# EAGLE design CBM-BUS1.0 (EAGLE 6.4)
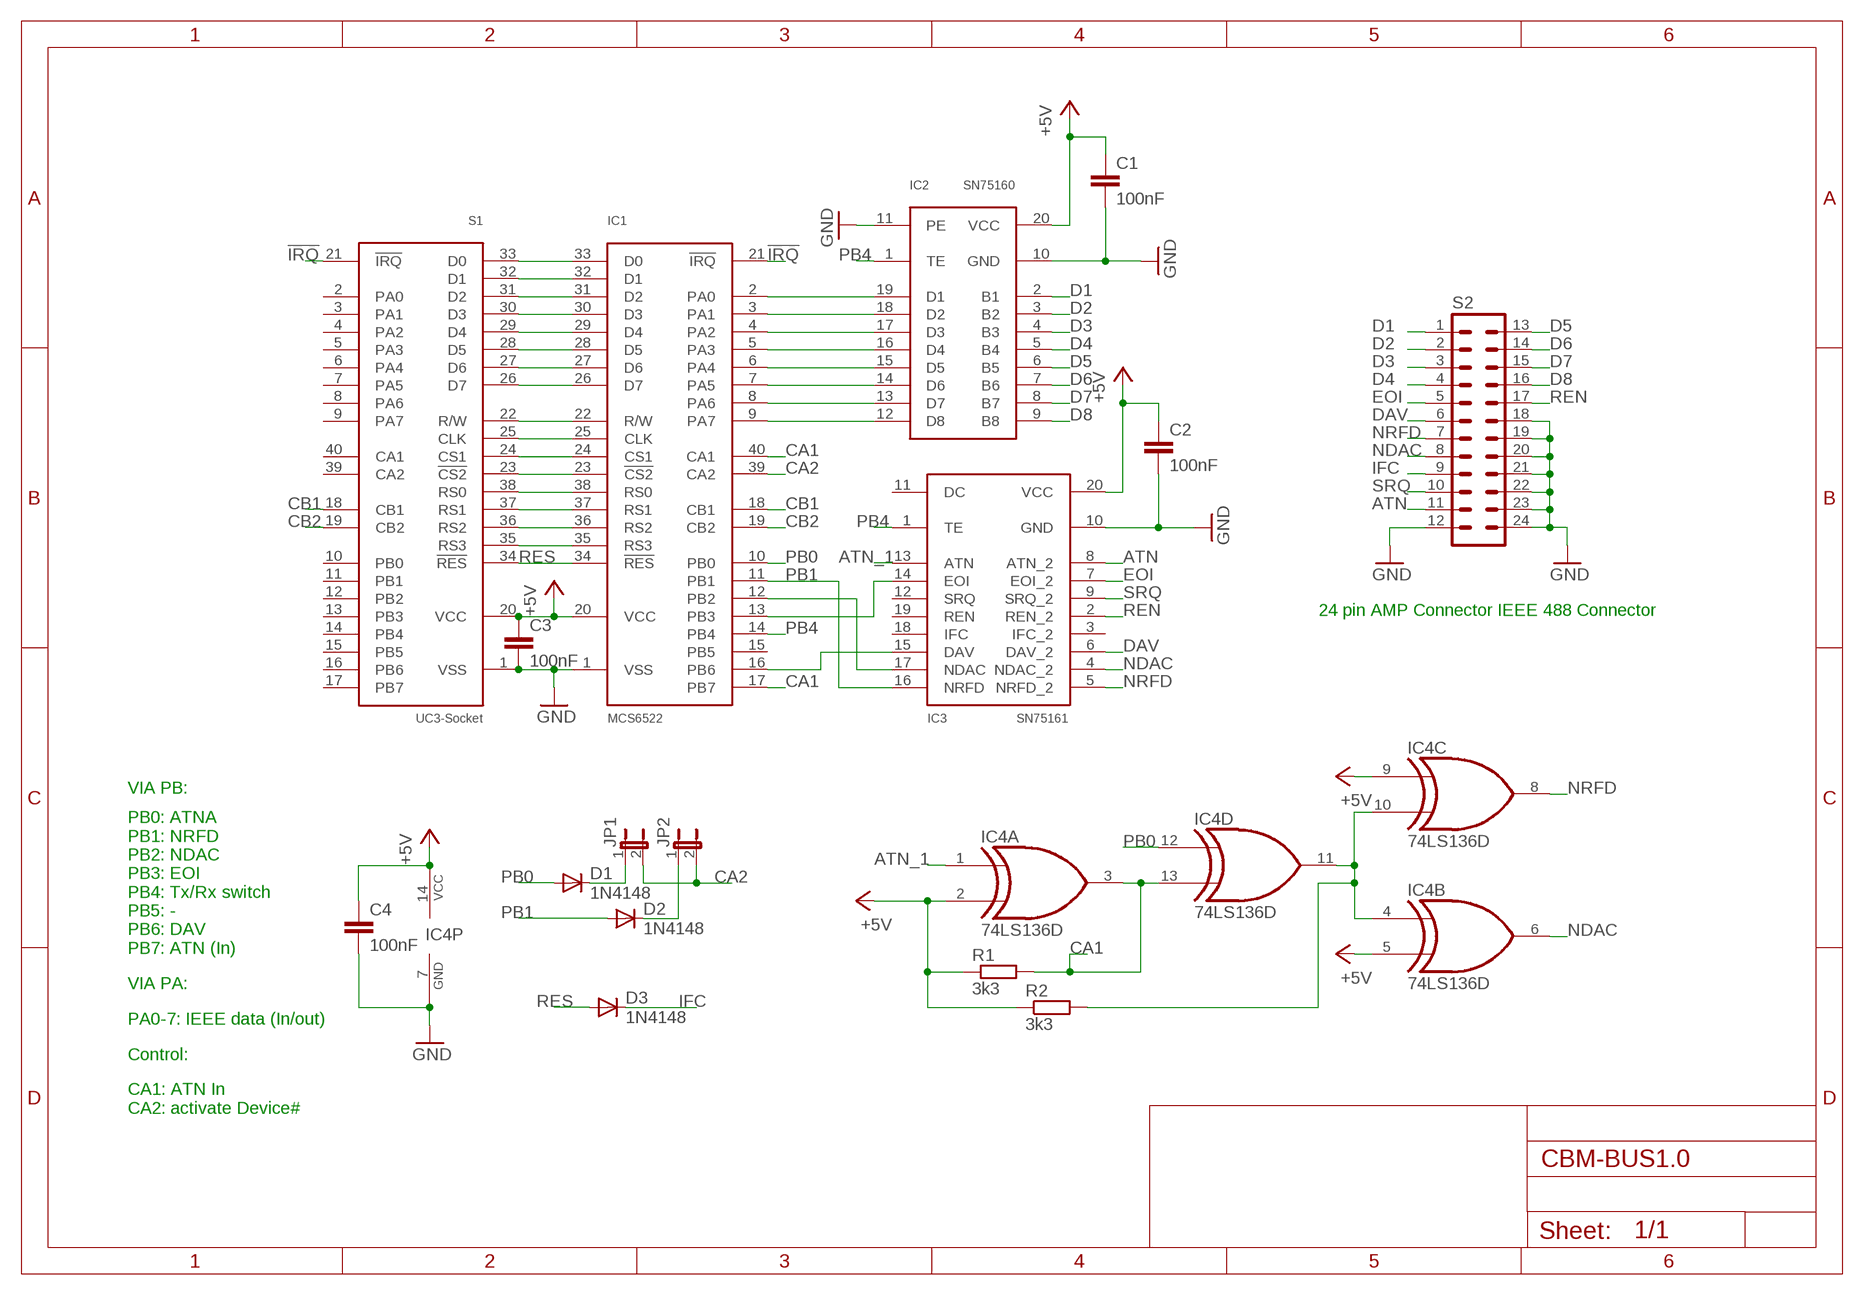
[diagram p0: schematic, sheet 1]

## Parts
C1  100nF  C-EU050-024X044  [C050-024X044]
C2  100nF  C-EU050-024X044  [C050-024X044]
C3  100nF  C-EU050-024X044  [C050-024X044]
C4  100nF  C-EU050-024X044  [C050-024X044]
D1  1N4148  1N4148DO35-10  [DO35-10]
D2  1N4148  1N4148DO35-10  [DO35-10]
D3  1N4148  1N4148DO35-10  [DO35-10]
IC1  MCS6522  [DIL40]
IC2  SN75160  [DIL20]
IC3  SN75161  [DIL20]
IC4  74LS136D  [DIL14]
JP1  JP1E  [JP1]
JP2  JP1E  [JP1]
R1  3k3  R-EU_0207/12  [0207/12]
R2  3k3  R-EU_0207/12  [0207/12]
S1  UC3-Socket  MCS6522  [DIL40]
S2  24PIN-SPECIAL  [24PIN-SPECIAL]

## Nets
!IRQ: IC1.21(!IRQ) S1.21(!IRQ)
+5V: C1.1 C2.1 C3.1 C4.1 IC1.20(VCC) IC2.20(VCC) IC3.20(VCC) IC4.2(A:I1) IC4.5(B:I1) IC4.9(C:I0) IC4.14(P:VCC) R1.1 R2.1 S1.20(VCC)
ATN: IC3.8(ATN_2) S2.11
ATN_1: IC3.13(ATN) IC4.1(A:I0)
CA1: IC1.17(PB7) IC1.40(CA1) IC4.3(A:O) IC4.13(D:I1) R1.2
CA2: IC1.39(CA2) JP1.2 JP2.2
CB1: IC1.18(CB1) S1.18(CB1)
CB2: IC1.19(CB2) S1.19(CB2)
D1: IC2.2(B1) S2.1
D2: IC2.3(B2) S2.2
D3: IC2.4(B3) S2.3
D4: IC2.5(B4) S2.4
D5: IC2.6(B5) S2.13
D6: IC2.7(B6) S2.14
D7: IC2.8(B7) S2.15
D8: IC2.9(B8) S2.16
DAV: IC3.6(DAV_2) S2.6
EOI: IC3.7(EOI_2) S2.5
GND: C1.2 C2.2 C3.2 C4.2 IC1.1(VSS) IC2.10(GND) IC2.11(PE) IC3.10(GND) IC4.7(P:GND) S1.1(VSS) S2.12 S2.18 S2.19 S2.20 S2.21 S2.22 S2.23 S2.24
IFC: D3.C S2.9
N$1: IC1.33(D0) S1.33(D0)
N$2: IC1.32(D1) S1.32(D1)
N$3: IC1.31(D2) S1.31(D2)
N$4: IC1.30(D3) S1.30(D3)
N$5: IC1.29(D4) S1.29(D4)
N$6: IC1.28(D5) S1.28(D5)
N$7: IC1.27(D6) S1.27(D6)
N$8: IC1.26(D7) S1.26(D7)
N$9: IC1.38(RS0) S1.38(RS0)
N$10: IC1.37(RS1) S1.37(RS1)
N$11: IC1.36(RS2) S1.36(RS2)
N$12: IC1.35(RS3) S1.35(RS3)
N$13: IC1.25(CLK) S1.25(CLK)
N$14: IC1.24(CS1) S1.24(CS1)
N$15: IC1.23(!CS2) S1.23(!CS2)
N$16: IC1.22(R/W) S1.22(R/W)
N$17: D1.C JP1.1
N$18: D2.C JP2.1
N$19: IC1.2(PA0) IC2.19(D1)
N$20: IC1.3(PA1) IC2.18(D2)
N$21: IC1.4(PA2) IC2.17(D3)
N$22: IC1.5(PA3) IC2.16(D4)
N$23: IC1.6(PA4) IC2.15(D5)
N$24: IC1.7(PA5) IC2.14(D6)
N$25: IC1.8(PA6) IC2.13(D7)
N$26: IC1.9(PA7) IC2.12(D8)
N$27: IC4.4(B:I0) IC4.10(C:I1) IC4.11(D:O) R2.2
N$28: IC1.12(PB2) IC3.17(NDAC)
N$29: IC1.13(PB3) IC3.14(EOI)
N$31: IC1.16(PB6) IC3.15(DAV)
NDAC: IC3.4(NDAC_2) IC4.6(B:O) S2.8
NRFD: IC3.5(NRFD_2) IC4.8(C:O) S2.7
PB0: D1.A IC1.10(PB0) IC4.12(D:I0)
PB1: D2.A IC1.11(PB1) IC3.16(NRFD)
PB4: IC1.14(PB4) IC2.1(TE) IC3.1(TE)
REN: IC3.2(REN_2) S2.17
RES: D3.A IC1.34(!RES) S1.34(!RES)
SRQ: IC3.9(SRQ_2) S2.10
Unconnected: IC1.15(PB5) IC3.3(IFC_2) IC3.11(DC) IC3.12(SRQ) IC3.18(IFC) IC3.19(REN) S1.2(PA0) S1.3(PA1) S1.4(PA2) S1.5(PA3) S1.6(PA4) S1.7(PA5) S1.8(PA6) S1.9(PA7) S1.10(PB0) S1.11(PB1) S1.12(PB2) S1.13(PB3) S1.14(PB4) S1.15(PB5) S1.16(PB6) S1.17(PB7) S1.39(CA2) S1.40(CA1)

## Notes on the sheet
- 24 pin AMP Connector IEEE 488 Connector
- VIA PB:
- PB0: ATNA
  PB1: NRFD
  PB2: NDAC
  PB3: EOI
  PB4: Tx/Rx switch
  PB5: -
  PB6: DAV
  PB7: ATN (In)
- VIA PA:
- PA0-7: IEEE data (In/out)
- Control:
- CA1: ATN In
  CA2: activate Device#

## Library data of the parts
C1-C4 = rcl:C-EU: CAPACITOR, European symbol
D1-D3 = diode:1N4148: DIODE
IC1 S1 = Nikon:MCS6522: MCS6522 - Versatile Interface Adapter Datasheet: link
IC2 = Nikon:SN75160: SN75160B Octal General-Purpose Interface Bus Transceiver Datasheet: link
IC3 = Nikon:SN75161: SN75161B Octal General-Purpose Interface Bus Transceivers Datasheet: link
IC4 = 74xx-us:74*136: Quad EXCLUSIV-OR/NOR (XOR/NOR) gate, open collector
JP1 JP2 = jumper:JP1E: JUMPER
R1 R2 = rcl:R-EU_: RESISTOR, European symbol
S2 = Nikon:24PIN-SPECIAL: PIN HEADER

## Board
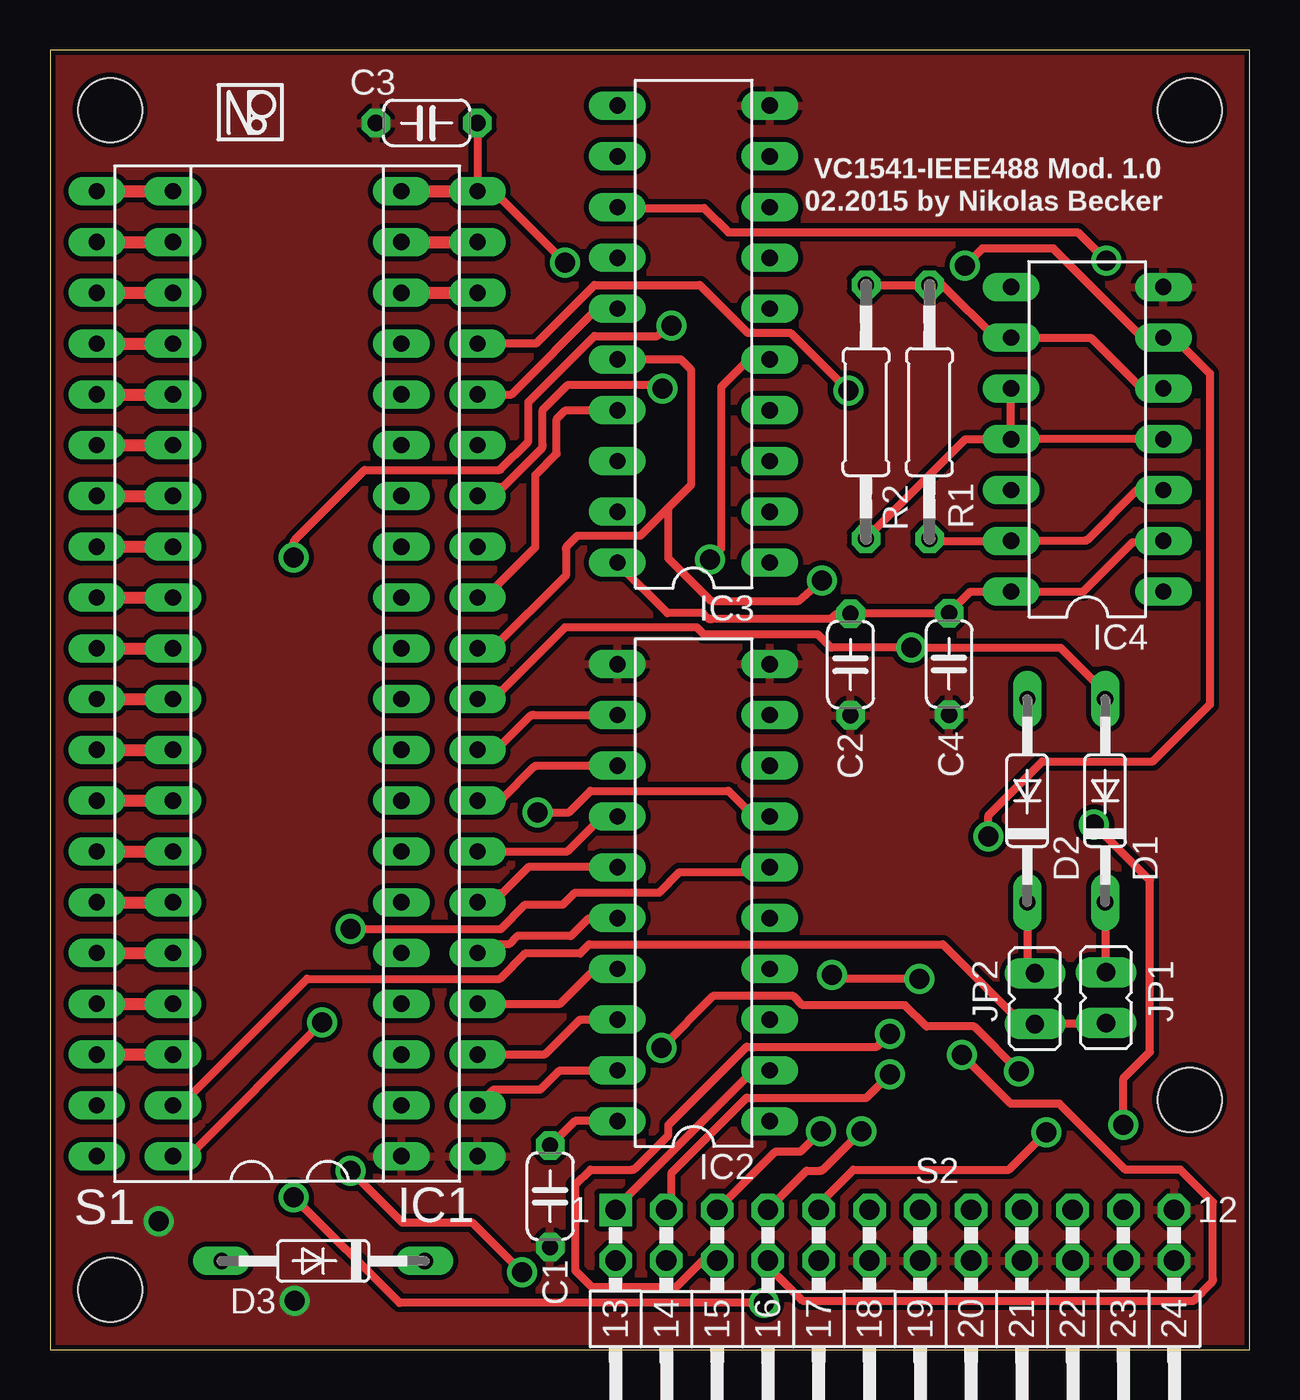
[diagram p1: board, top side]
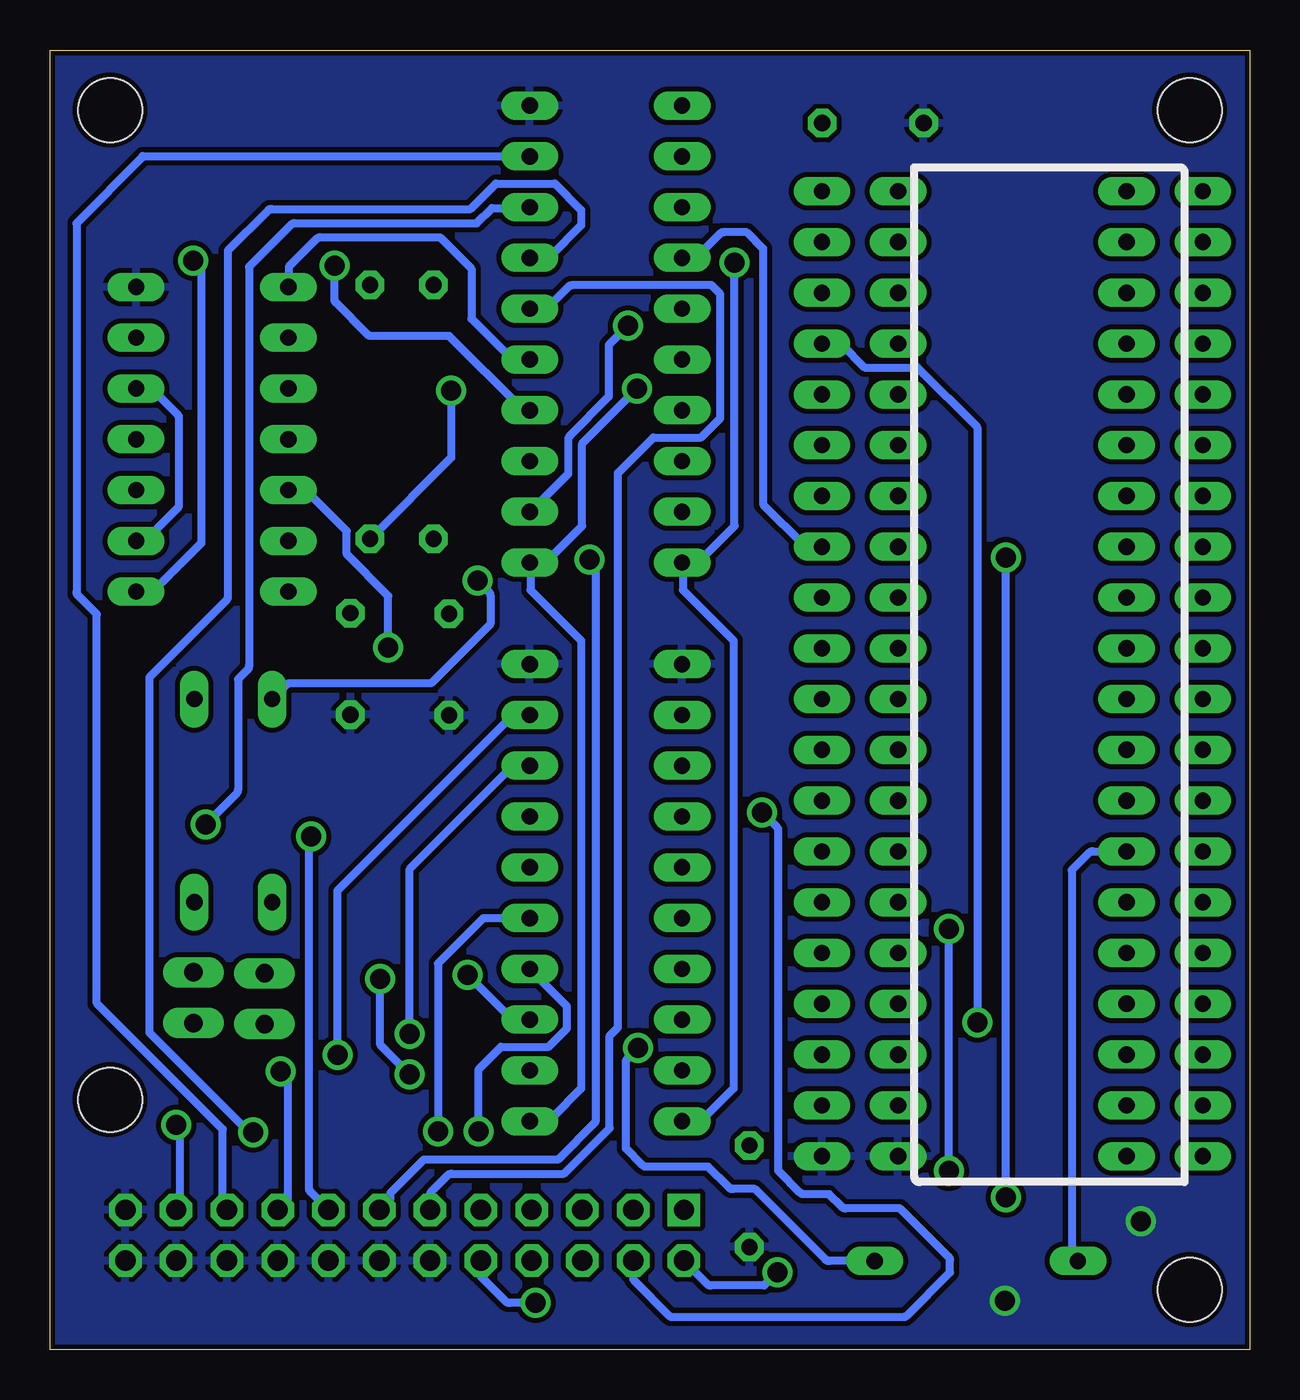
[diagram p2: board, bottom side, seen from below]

Size 60 x 65 mm. Coordinates in mm from the lower left corner, seen from the top.
Outline: 0,0 60,0 60,65 0,65 0,0
Copper layers (1*16): Top 0.035mm / dielectric 1.5mm / Bottom 0.035mm
Design rules "DFRobot_Eagle_Rule_v0.4 *": minimum track width 6mil, minimum drill 12mil, track to track 10mil, track to pad 10mil, pad to pad 10mil, via to via 10mil, smd to smd 6mil, copper to edge 10mil, drill to drill 10mil, minimum pad ring 12mil, minimum via ring 8mil, stop-mask expansion 2mil, vias tented up to drill 25mil, thermal gap 10mil
Holes 3.2 mm at 3,62 57,62 3,3 57,12.5

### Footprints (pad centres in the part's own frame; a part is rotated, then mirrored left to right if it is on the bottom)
C050-024X044 = drill 0.813 octagon: 1 -2.54,0; 2 2.54,0
DO35-10 = drill 0.813 long: A 5.08,0; C -5.08,0
DIL40 = drill 0.813 long: 1 -24.13,-7.62; 2 -21.59,-7.62; 3 -19.05,-7.62; 4 -16.51,-7.62; 5 -13.97,-7.62; 6 -11.43,-7.62; 7 -8.89,-7.62; 8 -6.35,-7.62; 9 -3.81,-7.62; 10 -1.27,-7.62; 11 1.27,-7.62; 12 3.81,-7.62; 13 6.35,-7.62; 14 8.89,-7.62; 15 11.43,-7.62; 16 13.97,-7.62; 17 16.51,-7.62; 18 19.05,-7.62; 19 21.59,-7.62; 20 24.13,-7.62; 21 24.13,7.62; 22 21.59,7.62; 23 19.05,7.62; 24 16.51,7.62; 25 13.97,7.62; 26 11.43,7.62; 27 8.89,7.62; 28 6.35,7.62; 29 3.81,7.62; 30 1.27,7.62; 31 -1.27,7.62; 32 -3.81,7.62; 33 -6.35,7.62; 34 -8.89,7.62; 35 -11.43,7.62; 36 -13.97,7.62; 37 -16.51,7.62; 38 -19.05,7.62; 39 -21.59,7.62; 40 -24.13,7.62
DIL20 = drill 0.813 long: 1 -11.43,-3.81; 2 -8.89,-3.81; 3 -6.35,-3.81; 4 -3.81,-3.81; 5 -1.27,-3.81; 6 1.27,-3.81; 7 3.81,-3.81; 8 6.35,-3.81; 9 8.89,-3.81; 10 11.43,-3.81; 11 11.43,3.81; 12 8.89,3.81; 13 6.35,3.81; 14 3.81,3.81; 15 1.27,3.81; 16 -1.27,3.81; 17 -3.81,3.81; 18 -6.35,3.81; 19 -8.89,3.81; 20 -11.43,3.81
DIL14 = drill 0.813 long: 1 -7.62,-3.81; 2 -5.08,-3.81; 3 -2.54,-3.81; 4 0,-3.81; 5 2.54,-3.81; 6 5.08,-3.81; 7 7.62,-3.81; 8 7.62,3.81; 9 5.08,3.81; 10 2.54,3.81; 11 0,3.81; 12 -2.54,3.81; 13 -5.08,3.81; 14 -7.62,3.81
JP1 = drill 0.914 long: 1 0,-1.27; 2 0,1.27
0207/12 = drill 0.813 octagon: 1 -6.35,0; 2 6.35,0
24PIN-SPECIAL = drill 1.016 square: 1 13.97,-1.27 | drill 1.016 octagon: 2 11.43,-1.27; 3 8.89,-1.27; 4 6.35,-1.27; 5 3.81,-1.27; 6 1.27,-1.27; 7 -1.27,-1.27; 8 -3.81,-1.27; 9 -6.35,-1.27; 10 -8.89,-1.27; 11 -11.43,-1.27; 12 -13.97,-1.27; 13 13.97,1.27; 14 11.43,1.27; 15 8.89,1.27; 16 6.35,1.27; 17 3.81,1.27; 18 1.27,1.27; 19 -1.27,1.27; 20 -3.81,1.27; 21 -6.35,1.27; 22 -8.89,1.27; 23 -11.43,1.27; 24 -13.97,1.27

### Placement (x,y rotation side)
C1  25.02,7.67 270 top
C2  40.04,34.26 270 top
C3  18.84,61.34 180 top
C4  44.97,34.29 270 top
D1  52.78,27.45 90 top
D2  48.89,27.45 90 top
D3  13.67,4.43 180 top
IC1  13.77,33.8 90 top
IC2  32.2,22.85 90 top
IC3  32.2,50.79 90 top
IC4  51.88,45.53 90 top
JP1  52.82,17.6 180 top
JP2  49.27,17.55 180 top
R1  43.99,46.9 270 top
R2  40.81,46.9 270 top
S1  9.96,33.8 90 top
S2  42.26,5.71 180 top
U$1  [NSYMB]  9.96,61.87 0 top

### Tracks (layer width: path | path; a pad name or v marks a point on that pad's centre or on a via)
!IRQ
  Top 0.61: S1.21 IC1.21
+5V  (via drill 1)
  Top 0.406: C1.1 25.04,10.21 26.26,11.43 28.35,11.43 IC2.20 | IC3.20 28.4,39.32 30.89,36.83 32.66,36.83 32.9,36.6 arc45 33.07,36.52 39.06,36.52 39.26,36.73 arc-45 39.44,36.8 C2.1 arc-45 40.12,36.83 C4.1 | IC4.2 55.63,40.39 54.15,40.39 51.68,37.91 IC4.14 46.05,37.91 C4.1 | R2.1 R1.1 44.65,53.24 47.28,50.61 IC4.9 51.95,50.61 arc-45 52.13,50.54 54.61,48.06 55.66,48.06 arc45 IC4.5 | v25.76,54.36 22.25,57.86 arc45 22.07,57.94 IC1.20 C3.1 | C4.1 arc-45 44.89,36.8
  Top 0.61: S1.20 IC1.20
  Bottom 0.406: IC2.20 28.35,11.43 27.28,11.43 27.28,11.58 25.81,13.06 25.81,35.46 28.35,38 28.35,39.32 IC3.20 28.14,39.37 27.58,39.37 25.76,41.2 v25.76,54.36 | IC4.2 55.36,40.45 arc-45 55.18,40.52 53.54,42.16 53.54,46.58 arc-45 53.62,46.76 54.91,48.06 55.66,48.06 arc45 IC4.5
ATN  (via drill 1)
  Top 0.406: v52.22,26.26 55.02,23.47 55.02,14.88 53.7,13.56 v53.7,11.23
  Bottom 0.406: v53.7,11.23 53.49,11.02 53.49,7.67 53.65,7.52 53.65,7.01 S2.11 | IC3.8 36.02,57.1 37.9,57.1 38.66,56.34 47.75,56.34 arc-45 47.93,56.26 50.04,54.15 50.04,34.19 arc45 50.11,34.01 50.6,33.53 50.6,27.99 arc45 50.67,27.82 v52.22,26.26
ATN_1  (via drill 1)
  Top 0.406: v52.83,54.46 51.41,55.88 33.93,55.88 32.72,57.1 28.4,57.1 IC3.13
  Bottom 0.406: v52.83,54.46 52.43,54.05 52.43,40.34 54.78,37.98 arc45 54.96,37.91 IC4.1
CA1  (via drill 1)
  Top 0.406: IC4.3 55.68,42.98 54.36,42.98 51.9,40.52 arc-45 51.72,40.45 IC4.13 44.19,40.45 arc-45 44.01,40.52 R1.2 | v13.61,16.36 7.01,9.75 arc-45 6.83,9.68 IC1.40 | v39.93,47.95 37.03,50.85 34.9,50.85 32.51,53.24 27.23,53.24 24.3,50.31 IC1.17 21.39,50.34
  Bottom 0.406: v13.61,16.36 13.61,46.13 16.61,49.12 19.25,49.12 20.42,50.29 arc-45 20.48,50.31 IC1.17 | v39.93,47.95 39.93,44.6 43.94,40.59 R1.2
CA2
  Top 0.406: JP1.2 52.32,16.31 49.78,16.31 JP2.2 49.58,16.31 48.62,16.31 44.65,20.27 26.98,20.27 26.52,19.81 23.77,19.81 22.5,18.54 12.85,18.54 6.53,12.21 IC1.39
CB1
  Top 0.61: S1.18 IC1.18
CB2
  Top 0.61: S1.19 IC1.19
D1
  Top 0.406: S2.1 arc45 28.3,7 28.3,7.06 35.12,13.89 arc-45 35.3,13.96 IC2.2
D2  (via drill 1)
  Top 0.406: v39.12,18.75 39.32,18.54 v43.48,18.54 | v42.01,13.77 40.84,12.6 34.85,12.6 31.09,8.84 31.09,7.35 arc-45 31.02,7.17 S2.2
  Bottom 0.406: v43.48,18.54 43.48,15.24 v42.01,13.77 | IC2.3 36.77,16.5 arc45 36.95,16.57 v39.12,18.75
D3  (via drill 1)
  Top 0.406: S2.3 36.22,9.83 arc-45 36.4,9.91 37.49,9.91 arc45 37.58,9.94 v38.56,10.92
  Bottom 0.406: v38.56,10.92 38.56,14.02 37.44,15.14 35.05,15.14 34.14,16.05 34.14,17.17 35.97,19 IC2.4
D4  (via drill 1)
  Top 0.406: S2.4 arc-45 35.92,7.02 37.85,8.94 38.5,8.94 arc45 38.68,9.02 v40.59,10.92
  Bottom 0.406: v40.59,10.92 40.59,19.3 38.31,21.58 IC2.5
D5  (via drill 1)
  Top 0.406: v15.04,21.03 22.55,21.03 23.77,22.25 25.65,22.25 26.26,22.86 30.48,22.86 31.5,23.88 35.76,23.88 35.97,24.08 IC2.6 | v15.04,8.94 17.63,6.35 21.13,6.35 v23.62,3.86
  Bottom 0.406: v15.04,8.94 v15.04,21.03 | v23.62,3.86 24.28,3.2 26.94,3.2 arc45 27.12,3.27 S2.13
D6  (via drill 1)
  Top 0.406: v24.38,26.87 25.96,26.87 27.03,27.94 33.93,27.94 35.14,26.73 arc45 35.32,26.66 IC2.7
  Bottom 0.406: S2.14 30.83,3.6 arc-45 30.76,3.42 29.03,1.7 arc-45 28.85,1.63 17.33,1.63 arc-45 17.15,1.7 14.99,3.86 14.99,4.47 arc-45 15.06,4.65 17.48,7.06 20.21,7.06 arc45 20.39,7.14 21.03,7.77 22.3,7.77 arc45 22.48,7.85 23.57,8.94 23.57,25.95 arc-45 23.65,26.14 v24.38,26.87
D7  (via drill 1)
  Top 0.406: v42.01,15.8 41.35,15.14 34.85,15.14 30.94,11.23 30.94,10.72 29.28,9.07 arc-45 29.11,8.99 27.03,8.99 26.26,8.23 26.26,3.96 27.08,3.15 31.34,3.15 32.61,4.42 33.33,4.42 S2.15
  Bottom 0.406: v42.01,15.8 42.01,24.03 37.08,28.96 37.08,29.16 36.02,29.16 IC2.8
D8  (via drill 1)
  Top 0.406: v45.62,14.73 48.06,12.29 50.49,12.29 53.8,8.99 56.54,8.99 58.17,7.37 58.17,3.51 arc-45 58.09,3.33 57.2,2.44 37.64,2.44 35.92,4.17 35.92,4.42 S2.16
  Bottom 0.406: v45.62,14.73 45.62,22.96 37.08,31.5 37.08,31.7 36.02,31.7 IC2.9
DAV
  Bottom 0.406: S2.6 40.99,7.72 arc45 40.92,7.9 40.1,8.71 arc45 39.92,8.79 34.29,8.79 32,11.07 32,15.7 31.6,16.1 31.6,43.84 29.82,45.62 27.43,45.62 26.47,46.58 26.47,52.78 26.92,53.24 33.88,53.24 arc-45 34.06,53.16 35.15,52.07 35.98,52.07 arc-45 IC3.6
EOI  (via drill 1)
  Top 0.406: v49.84,10.87 47.95,8.99 40.18,8.99 38.46,7.26 38.46,7.01 S2.5
  Bottom 0.406: IC3.7 35.17,54.6 arc-45 34.99,54.67 33.43,56.24 33.43,57 34.75,58.32 37.69,58.32 38.96,57.05 48.92,57.05 arc-45 49.1,56.97 51.1,54.97 51.1,37.65 arc45 51.18,37.47 55.02,33.63 55.02,15.85 50.04,10.87 v49.84,10.87
GND  (via drill 1)
  other vias: 5.44,6.4 12.24,2.44
  pour Bottom: 0,0 60,0 60,65 0,65
  pour Top: 0,0 60,0 60,65 0,65
IFC  (via drill 1)
  Top 0.406: v30.58,15.09 33.17,17.68 37.19,17.68 37.64,17.22 42.77,17.22 43.84,16.15 46.23,16.15 v48.46,13.92
  Bottom 0.406: D3.C 21.03,4.43 arc45 21.21,4.5 24.74,8.03 25.85,8.03 arc45 26.03,8.1 27.08,9.14 30.17,9.14 arc45 30.35,9.22 31.19,10.06 31.19,14.37 arc45 31.12,14.55 v30.58,15.09 | v48.46,13.92 48.18,13.64 arc45 48.11,13.46 48.11,7.59 arc45 48.18,7.41 S2.9
N$1
  Top 0.61: S1.33 IC1.33
N$2
  Top 0.61: S1.32 IC1.32
N$3
  Top 0.61: S1.31 IC1.31
N$4
  Top 0.61: S1.30 IC1.30
N$5
  Top 0.61: S1.29 IC1.29
N$6
  Top 0.61: S1.28 IC1.28
N$7
  Top 0.61: S1.27 IC1.27
N$8
  Top 0.61: S1.26 IC1.26
N$9
  Top 0.61: S1.38 IC1.38
N$10
  Top 0.61: S1.37 IC1.37
N$11
  Top 0.61: S1.36 IC1.36
N$12
  Top 0.61: S1.35 IC1.35
N$13
  Top 0.61: S1.25 IC1.25
N$14
  Top 0.61: S1.24 IC1.24
N$15
  Top 0.61: S1.23 IC1.23
N$16
  Top 0.61: S1.22 IC1.22
N$17
  Top 0.406: D1.C 52.78,18.91 JP1.1
N$18
  Top 0.406: D2.C 48.89,19.2 JP2.1
N$19
  Top 0.406: IC1.2 22.1,12.93 arc-45 22.28,13.01 24.54,13.01 25.42,13.89 arc-45 25.6,13.96 IC2.19
N$20
  Top 0.406: IC1.3 24.66,14.76 arc45 24.84,14.83 26.43,16.43 arc-45 26.61,16.5 IC2.18
N$21
  Top 0.406: IC1.4 25.52,17.3 27.27,19.04 IC2.17
N$22
  Top 0.406: IC1.5 21.39,19.86 21.79,20.27 22.96,20.27 23.37,20.68 26.06,20.68 26.92,21.54 28.35,21.54 IC2.16
N$23
  Top 0.406: IC1.6 21.39,22.4 21.79,22.81 22.61,22.81 23.93,24.13 28.35,24.13 IC2.15
N$24
  Top 0.406: IC1.7 25.88,24.91 27.63,26.66 IC2.14
N$25
  Top 0.406: IC1.8 22.42,27.45 arc45 22.6,27.53 24.2,29.13 arc-45 24.38,29.2 IC2.13
N$26
  Top 0.406: IC1.9 22.22,30 arc45 22.4,30.07 24,31.67 arc-45 24.18,31.74 IC2.12
N$27
  Top 0.406: R2.2 40.84,40.59 45.72,45.47 arc-45 45.88,45.53 IC4.11 | IC4.4 IC4.11 | IC4.11 IC4.10
N$28
  Top 0.406: IC1.12 21.77,37.62 24.28,40.13 24.28,43.74 25.35,44.81 25.35,46.53 25.8,46.98 IC3.17
N$29
  Bottom 0.406: IC3.14 27.71,54.6 arc-45 27.69,54.61 26.49,55.81 arc45 26.31,55.88 25.15,55.88 24.33,55.07 24.33,42.27 22.3,40.23 arc-45 22.12,40.16 IC1.13
N$31
  Top 0.406: IC3.15 27.37,52.06 23.09,47.77 IC1.16
NDAC  (via drill 1)
  Top 0.406: v45.77,54.2 46.63,55.07 50.19,55.07 54.61,50.65 55.68,50.65 IC4.6 56.22,50.61 58.01,48.82 58.01,32.26 55.17,29.41 49.63,29.41 46.94,26.72 v46.94,25.65
  Bottom 0.406: S2.8 46.97,7.88 arc45 47.04,8.06 47.04,25.45 arc45 46.97,25.63 v46.94,25.65 | IC3.4 36.21,46.98 arc45 36.39,47.05 40.03,50.7 43.94,50.7 arc45 44.12,50.77 45.7,52.35 arc45 45.77,52.53 v45.77,54.2
NRFD  (via drill 1)
  Top 0.406: v33.02,39.52 33.58,40.08 33.58,48.16 34.94,49.52 IC3.5 35.97,49.48
  Bottom 0.406: v33.02,39.52 32.72,39.22 32.72,11.38 34.59,9.5 41.3,9.5 42.98,7.82 42.98,7.52 43.48,7.01 S2.7 | IC4.8 arc-45 48.06,53.18 48.06,54.15 46.66,55.55 arc45 46.48,55.63 40.49,55.63 38.91,54.05 38.91,51.56 36.95,49.59 arc-45 36.77,49.52 IC3.5
PB0  (via drill 1)
  Top 0.406: D1.A 52.78,32.87 50.55,35.1 v43.08,35.1 39.06,35.1 38.41,35.76 32.72,35.76 32.36,36.12 25.76,36.12 22.61,32.97 21.79,32.97 21.39,32.56 IC1.10
  Bottom 0.406: v43.08,35.1 43.08,37.69 45.16,39.78 45.16,40.95 46.99,42.77 46.99,42.98 48.06,42.98 IC4.12
PB1  (via drill 1)
  Top 0.406: 21.39,35.05 22.15,35.05 25.81,38.71 25.81,40.03 arc-45 25.88,40.21 26.36,40.69 29.52,40.69 30.89,42.06 | 21.39,35.05 21.34,35.05 | 30.89,42.06 32.05,43.23 32.05,49.02 31.56,49.52 IC3.16 | v38.61,38.46 37.44,37.44 33.07,37.44 30.94,39.57 30.94,42.01 30.89,42.06 | IC1.11 21.39,35.05
  Bottom 0.406: D2.A 48.17,33.25 arc45 47.99,33.33 40.95,33.33 37.97,36.3 37.97,37.71 arc-45 38.05,37.89 v38.61,38.46
PB4  (via drill 1)
  Top 0.406: IC1.14 21.39,42.72 21.79,43.13 22.66,43.13 24.56,45.04 arc45 24.64,45.22 24.64,46.99 25.83,48.19 arc-45 26.01,48.26 30.32,48.26 arc-45 30.5,48.19 v30.63,48.06
  Bottom 0.406: IC2.1 35.97,11.43 34.9,11.43 34.9,11.58 33.43,13.06 33.43,35.46 35.97,38 35.97,39.32 IC3.1 35.76,39.37 35.2,39.37 33.38,41.2 33.38,45.31 v30.63,48.06
REN  (via drill 1)
  Top 0.406: v31.09,51.21 30.38,50.7 27.23,50.7 23.93,47.4 23.93,45.41 22.54,44.03 arc-45 22.45,43.99 15.75,43.99 12.27,40.51 arc45 12.19,40.33 v12.19,39.62 | v12.19,7.62 17.48,2.34 v35.71,2.34
  Bottom 0.406: v31.09,51.21 32.05,50.24 32.05,47.65 34.04,45.67 34.04,45.62 34.09,45.57 34.09,43.79 35.97,41.91 IC3.2 | v12.19,7.62 v12.19,39.62 | v35.71,2.34 37.03,2.34 arc45 37.21,2.41 38.46,3.66 38.46,4.43 arc45 S2.17
RES
  Top 0.61: S1.34 IC1.34
  Bottom 0.406: D3.A 8.82,4.66 arc45 8.89,4.84 8.89,23.98 8.03,24.84 arc45 7.85,24.91 IC1.34
SRQ
  Bottom 0.406: IC3.9 55.37,59.69 arc45 55.41,59.6 58.67,56.34 58.67,37.9 arc-45 58.6,37.72 57.66,36.78 57.66,17.32 51.36,11.02 51.36,7.21 51.16,7.01 S2.10

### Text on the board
tNames: VC1541-IEEE488 Mod. 1.0 | 02.2015 by Nikolas Becker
